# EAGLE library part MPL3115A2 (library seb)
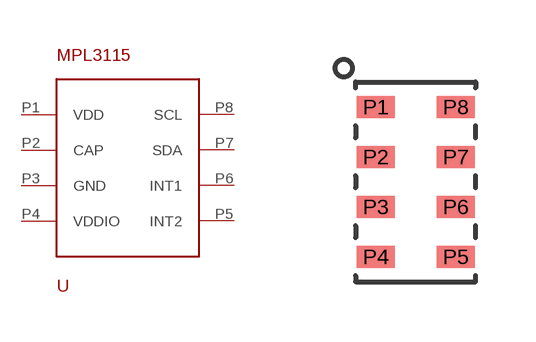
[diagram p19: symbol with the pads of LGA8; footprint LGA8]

Designator prefix -

## MPL3115A2  [LGA8]
P1  VDD
P2  CAP
P3  GND
P4  VDDIO
P5  INT2
P6  INT1
P7  SDA
P8  SCL

## Footprint LGA8 (pad centres in mm)
smd 0.95 x 0.55: P1 -1,1.875; P2 -1,0.625; P3 -1,-0.625; P4 -1,-1.875; P5 1,-1.875; P6 1,-0.625; P7 1,0.625; P8 1,1.875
